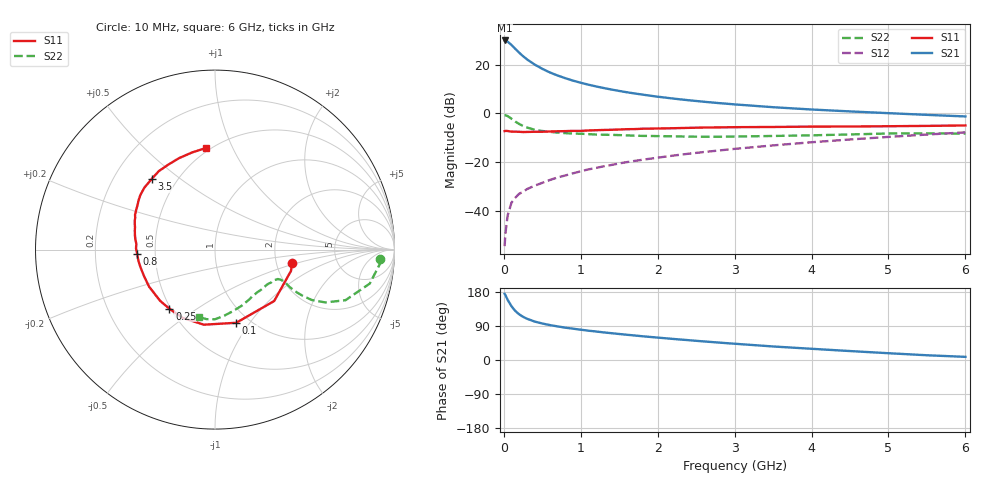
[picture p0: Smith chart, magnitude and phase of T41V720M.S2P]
! Infineon Technologies  Discrete & RF Semiconductors
! BFR182T
! Si NPN RF Bipolar Junction Transistor in SC75
! VCE = 1.75 V  IC = 20 mA
! Common Emitter S-Parameters:  October  1999
# GHz  S  MA  R  50
!  f  S11  S21  S12  S22
! GHz  MAG  ANG  MAG  ANG  MAG  ANG  MAG  ANG
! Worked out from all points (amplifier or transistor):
!   36 points, 10 MHz to 6 GHz, reference 50 ohm
!   highest |S21| = 29.9 dB at 10 MHz (marker M1)
!   |S21| within 3 dB of that: start of sweep to 134.9 MHz
!   unconditionally stable (mu >= 1): start of sweep to 10.51 MHz; 452.5 MHz to 4.129 GHz
!   at 250 MHz: K = 0.77, MSG = 27.8 dB, |S12| = -32.2 dB
!   at 1.4 GHz: K = 1.22, MAG = 12.6 dB, |S12| = -21.1 dB
!   at 6 GHz: K = 0.89, MSG = 3.3 dB, |S12| = -7.7 dB
!   S11 on the Smith chart (normalised r, x): 10 MHz: 2.45, -0.44; 100 MHz: 0.87, -0.86; 250 MHz: 0.49, -0.39; 800 MHz: 0.39, -0.02; 3.5 GHz: 0.36, +0.40; 6 GHz: 0.47, +0.79
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0.01  0.4351 -9.7  31.43 174.6  0.0019 86.1  0.9205 -3.3
0.02  0.4398 -15.6  31.41 171.3  0.0034 86.1  0.9215 -5.1
0.05  0.4368 -41.0  29.69 158.6  0.0082 81.4  0.8825 -12.4
0.1  0.4245 -73.8  25.3 141.7  0.0149 68.3  0.7798 -21.2
0.15  0.423 -98.4  21.04 129.2  0.0188 62.4  0.681 -25.6
0.2  0.4211 -115.3  17.61 120.4  0.0226 60.5  0.6084 -27.5
0.25  0.4158 -127.7  14.95 114.0  0.0246 59.4  0.5531 -27.8
0.3  0.4183 -137.0  12.91 108.9  0.0281 61.2  0.516 -27.6
0.4  0.4214 -150.7  10.09 101.5  0.033 61.5  0.4642 -26.6
0.5  0.4222 -159.7  8.237 96.3  0.0378 64.4  0.4374 -25.3
0.6  0.4269 -166.8  6.918 92.1  0.0433 66.0  0.4196 -24.9
0.7  0.4315 -172.0  5.996 88.6  0.0488 67.8  0.4048 -24.6
0.8  0.4343 -176.9  5.283 85.3  0.0536 68.0  0.395 -24.8
0.9  0.4401 179.1  4.708 82.6  0.0593 69.7  0.3862 -25.1
1.1  0.4483 172.2  3.894 77.3  0.0714 70.7  0.3767 -26.5
1.3  0.4592 166.6  3.322 72.8  0.0827 71.4  0.3661 -28.5
1.6  0.476 159.9  2.723 66.6  0.1006 71.5  0.3549 -32.0
2.2  0.4981 150.0  2.023 55.6  0.1367 70.7  0.3403 -41.3
3.5  0.5286 131.8  1.344 35.7  0.2214 66.1  0.3457 -64.0
4.5  0.5401 119.0  1.102 23.6  0.2928 60.2  0.3714 -81.8
5.5  0.5563 103.1  0.936 12.5  0.3698 53.1  0.3904 -96.9
6  0.5679 95.3  0.869 8.3  0.4101 48.7  0.3859 -103.4
